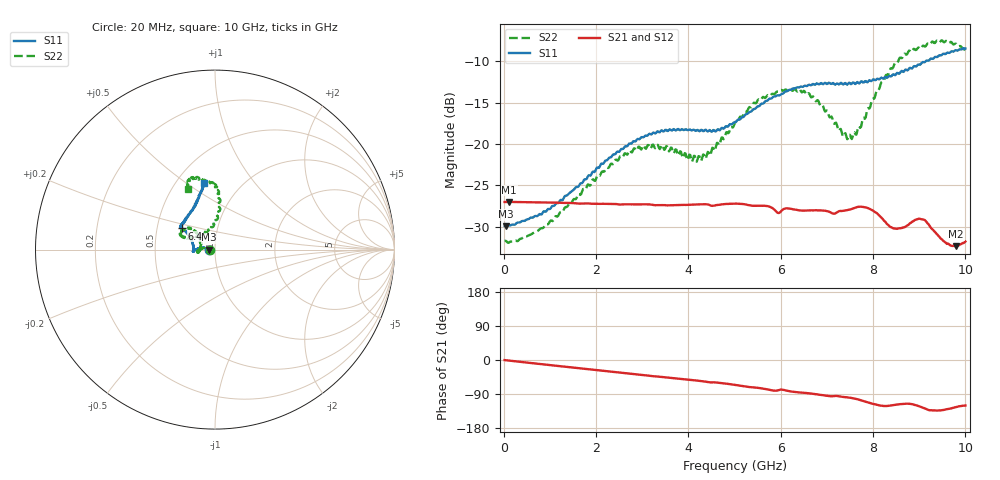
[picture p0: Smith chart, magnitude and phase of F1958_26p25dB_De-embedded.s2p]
! Integrated Device Technology
! Corporate Headquarters
! 6024 Silver Creek Valley Road
! San Jose, CA 95138  USA
! Phone:  1-408-284-8200
! Toll Free:  1-800-223-1366
! Webpage:  http://www.idt.com/
! Timing and RF Division
! 515 Groton Road, Suite 102
! Westford, MA 01886-6024
! Device:  F1958
! Description: 7-bit 0.25 dB Digital Step Attenuator
! Frequency:  0.001 -  6.000 GHz
! Package:  4x4 mm Thin QFN Plastic Package: 24 pin
! Ports:  2 RF, 12 DC
!  Pin  1  = D0
!  Pin  2  = VDD
!  Pin  3  = VMODE
!  Pin  4  = GND
!  Pin  5  = RF1  =  Port 1
!  Pin  6  = GND
!  Pin  7  = GND
!  Pin  8  = GND
!  Pin  9  = GND
!  Pin 10  = GND
!  Pin 11  = GND
!  Pin 12  = GND
!  Pin 13  = GND
!  Pin 14  = RF2  =  Port 2
!  Pin 15  = GND
!  Pin 16  = LE
!  Pin 17  = CLK
!  Pin 18  = DATA
!  Pin 19  = D6
!  Pin 20  = D5
!  Pin 21  = D4
!  Pin 22  = D3
!  Pin 23  = D2
!  Pin 24  = D1
! State:  105
! Atten State:  26.25 dB
! Voltage:  +3.30 Volts
! Current:  0.259 mA
! Data:  The device was measured on a F1958 evaluation board which has
!  individual transmission lines to the RF pins.  Data was collected
!  using a calibrated network analyzer.  The evaluation board was
!  de-embedded using Automatic Fixture Removal (AFR).
!  The reference plane is the edge of the package pin.
! Misc:
!  Action Tracker AT0419
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# GHz S dB R 50
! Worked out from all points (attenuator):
!   500 points, 20 MHz to 10 GHz, reference 50 ohm
!   highest |S21| = -26.99 dB at 120 MHz (marker M1); lowest = -32.3 dB at 9.8 GHz (marker M2)
!   lowest |S11| = -29.9 dB at 40 MHz (marker M3), VSWR 1.07, Z = 46.9 - j0.0439 ohm
!   |S11| at or under -10 dB: start of sweep to 9.137 GHz
!   |S22| runs from -31.9 to -7.5 dB; largest |S21 - S12| = 0.00031
!   S11 on the Smith chart (normalised r, x): 20 MHz: 0.94, -0.00; 6.4 GHz: 0.67, +0.17; 10 GHz: 0.68, +0.59
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0.02  -29.92 -178.9  -27.00 -0.3  -27.00 -0.2  -31.72 -178.9
0.04  -29.95 -179.2  -27.00 -0.5  -26.99 -0.5  -31.69 -178.5
0.12  -29.83 178.9  -26.99 -1.6  -26.99 -1.6  -31.89 178.8
0.84  -28.35 171.1  -27.06 -11.3  -27.05 -11.2  -30.17 172.2
1.7  -24.72 171.0  -27.19 -22.4  -27.18 -22.3  -25.69 171.1
2.62  -20.32 177.0  -27.28 -34.1  -27.27 -34.2  -21.11 -179.8
3.36  -18.56 -175.8  -27.38 -44.0  -27.38 -44.1  -20.41 -169.9
4.24  -18.45 -179.2  -27.29 -55.0  -27.30 -55.1  -21.49 168.4
4.5  -18.51 174.9  -27.46 -59.1  -27.46 -59.1  -20.84 151.0
5.02  -17.37 160.6  -27.19 -66.0  -27.20 -66.0  -17.30 138.0
5.58  -15.13 150.4  -27.46 -74.7  -27.47 -74.7  -14.59 139.7
6.4  -13.15 147.6  -28.01 -85.5  -28.03 -85.5  -13.39 155.4
6.68  -12.80 146.5  -28.00 -88.8  -28.03 -88.8  -14.31 157.3
7.5  -12.63 138.1  -27.92 -99.5  -27.92 -99.4  -18.87 119.3
7.68  -12.58 135.1  -27.59 -104.2  -27.59 -104.1  -17.92 99.3
7.92  -12.27 128.8  -27.81 -113.1  -27.80 -113.1  -15.71 88.2
8.34  -11.77 118.7  -29.83 -120.9  -29.83 -121.0  -11.45 83.8
8.66  -11.28 113.0  -30.06 -115.8  -30.12 -115.8  -9.25 87.5
9.1  -10.11 106.9  -29.15 -126.8  -29.15 -126.8  -8.11 100.1
9.56  -9.12 101.4  -31.87 -130.8  -31.91 -130.8  -7.61 108.4
9.8  -8.66 100.5  -32.34 -124.1  -32.37 -124.3  -7.87 112.5
10  -8.45 99.6  -31.78 -120.1  -31.83 -120.1  -8.63 113.6
